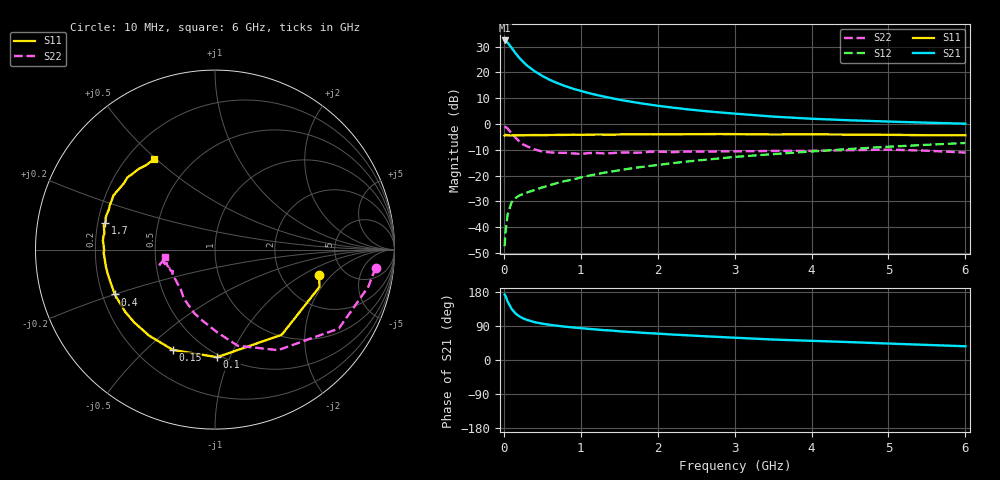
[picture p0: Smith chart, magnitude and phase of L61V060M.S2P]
!  INFINEON TECHNOLOGIES Small Signal Semiconductors
! BFR380L3 , Si-NPN RF-Transistor in TSLP-3-1
!  Vce=1 V,  Ic=60 mA
! Common Emitter S-Parameters:  07. March 2005
#  GHz  S  MA  R  50
! f  S11  S21  S12  S22
! GHz  Mag  Ang  Mag  Ang  Mag  Ang  Mag  Ang
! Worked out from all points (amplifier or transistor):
!   36 points, 10 MHz to 6 GHz, reference 50 ohm
!   highest |S21| = 32.4 dB at 10 MHz (marker M1)
!   |S21| within 3 dB of that: start of sweep to 104 MHz
!   unconditionally stable (mu >= 1): 1.107 GHz to end of sweep
!   at 250 MHz: K = 0.53, MSG = 25.6 dB, |S12| = -27.1 dB
!   at 1.4 GHz: K = 1.04, MAG = 13.0 dB, |S12| = -18.4 dB
!   at 6 GHz: K = 1.00, MAG = 3.3 dB, |S12| = -7.3 dB
!   S11 on the Smith chart (normalised r, x): 10 MHz: 3.28, -1.45; 100 MHz: 0.48, -0.90; 150 MHz: 0.34, -0.61; 400 MHz: 0.25, -0.20; 1.7 GHz: 0.23, +0.11; 6 GHz: 0.31, +0.49
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0.01  0.5978 -13.7  41.69 172.8  0.0043 70.4  0.9002 -6.5
0.02  0.6182 -19.6  40.99 169.4  0.0077 76.4  0.879 -13.6
0.05  0.6028 -51.9  37.75 153.9  0.0178 67.7  0.8183 -32.5
0.1  0.5997 -88.9  30.07 135.3  0.0302 56.0  0.6613 -57.9
0.15  0.6063 -112.9  23.8 123.1  0.0366 49.1  0.5504 -76.7
0.2  0.6039 -127.4  19.27 115.3  0.0412 48.0  0.4621 -88.3
0.25  0.6059 -138.0  16.12 109.9  0.044 46.6  0.4015 -100.2
0.3  0.6087 -145.2  13.7 105.8  0.047 47.3  0.3722 -108.2
0.4  0.6117 -155.9  10.57 99.8  0.0529 49.7  0.3227 -122.6
0.5  0.6101 -162.9  8.571 95.9  0.0591 52.1  0.2929 -130.5
0.6  0.6132 -167.7  7.149 92.7  0.0656 54.2  0.2828 -137.1
0.7  0.6154 -171.3  6.186 90.2  0.0723 56.4  0.2763 -143.2
0.9  0.621 -178.3  4.832 85.9  0.0846 59.4  0.2701 -151.8
1.1  0.6216 177.6  3.998 82.2  0.0997 61.4  0.2738 -154.9
1.4  0.6223 171.7  3.177 77.7  0.12 63.0  0.2731 -159.4
1.7  0.629 166.4  2.64 73.3  0.1413 63.7  0.2783 -164.3
2.2  0.6321 159.6  2.078 67.1  0.1752 63.9  0.2856 -164.5
2.8  0.6409 152.0  1.684 60.8  0.2157 63.7  0.2956 -167.6
3.5  0.6276 144.0  1.395 54.0  0.2611 61.3  0.3015 -166.4
4.5  0.6245 137.6  1.183 47.2  0.3292 59.0  0.3115 -165.6
5.5  0.607 129.2  1.063 39.8  0.3962 54.4  0.3043 -166.7
6  0.6075 124.2  1.017 36.2  0.4299 51.9  0.2801 -171.4
